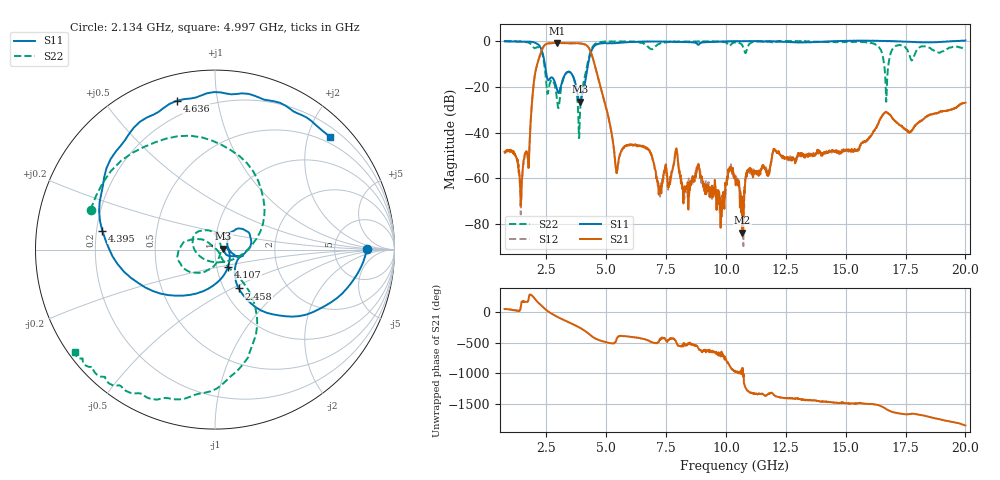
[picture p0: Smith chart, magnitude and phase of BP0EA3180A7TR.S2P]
! s2p File.  Ports: 1,3
# MHz S DB R 50
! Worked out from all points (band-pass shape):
!   1601 points, 750 MHz to 20 GHz, reference 50 ohm
!   highest |S21| = -0.86 dB at 2.928 GHz (marker M1); lowest = -83.6 dB at 10.69 GHz (marker M2)
!   |S21| within 3 dB of the highest: 2.31 GHz to 4.31 GHz (2 GHz wide, 60.4 % of centre)
!   lowest |S11| = -26.5 dB at 3.902 GHz (marker M3), VSWR 1.10, Z = 54.9 + j0.596 ohm
!   |S11| at or under -10 dB: 2.429 GHz to 4.242 GHz (1.812 GHz wide, 54.3 % of centre)
!   |S22| runs from -42.4 to 0.0 dB; largest |S21 - S12| = 0.01
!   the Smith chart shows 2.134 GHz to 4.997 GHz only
!   S11 on the Smith chart (normalised r, x): 2.134 GHz: 12, +0; 2.458 GHz: 1.17, -0.54; 4.107 GHz: 1.14, -0.22; 4.395 GHz: 0.22, +0.08; 4.636 GHz: 0.12, +0.77; 4.997 GHz: 0.38, +2.41
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750  -0.16 136.4  -48.37 54.8  -48.52 56.8  -0.19 159.3
1459.84  -0.30 82.4  -63.61 174.3  -62.65 176.8  -0.32 119.0
1868.91  -0.43 39.5  -30.29 -77.4  -30.28 -78.1  -1.60 23.3
2133.59  -1.45 0.1  -9.37 165.8  -9.37 165.3  -2.75 162.2
2458.44  -11.92 -58.6  -1.51 48.4  -1.53 47.9  -14.58 1.2
2927.66  -20.82 -9.3  -0.86 -68.8  -0.91 -69.0  -24.67 71.4
3902.19  -26.48 6.5  -1.12 105.2  -1.15 105.0  -30.71 -37.1
3962.34  -24.72 11.0  -1.19 91.7  -1.20 91.5  -23.55 -53.0
4106.72  -18.47 -52.2  -1.57 56.0  -1.57 55.8  -15.60 -49.9
4395.47  -3.92 170.4  -6.20 -32.2  -6.17 -32.9  -3.12 -81.2
4636.09  -1.35 104.3  -15.26 -85.9  -15.36 -86.2  -0.89 -117.2
4997.03  -0.95 44.3  -29.54 -128.7  -29.62 -129.0  -0.26 -143.8
5430.16  -0.93 -14.6  -57.72 -71.1  -57.57 -74.3  -0.25 -172.1
6669.38  -0.33 -94.2  -46.95 -88.3  -46.88 -89.0  -1.79 105.5
7174.69  -0.27 -106.8  -62.05 -121.3  -62.47 -134.2  -1.38 -87.2
10375  -0.10 121.2  -59.50 121.9  -61.45 104.9  -0.74 145.9
10687.81  -0.08 118.2  -83.64 171.5  -69.41 77.2  -2.14 130.8
13587.34  -0.57 37.1  -49.72 -1.1  -49.44 -3.3  -0.25 134.7
16330.47  0.03 17.3  -36.63 -76.2  -36.78 -76.2  -2.05 38.6
16799.69  -0.13 16.8  -31.97 -165.3  -31.82 -165.5  -9.20 150.8
18760.78  -0.60 -51.6  -31.58 62.9  -31.56 63.1  -4.86 6.1
20000  0.18 -75.8  -26.94 -51.2  -26.91 -50.2  -4.07 164.3
